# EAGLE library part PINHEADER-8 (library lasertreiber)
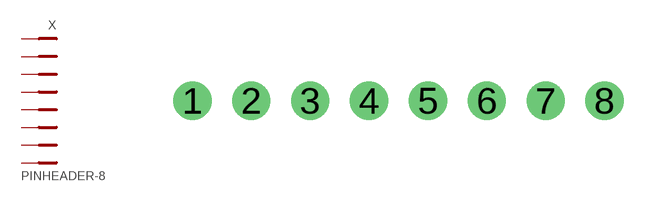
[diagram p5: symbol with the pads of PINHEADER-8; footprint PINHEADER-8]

Designator prefix X

## PINHEADER-8  [PINHEADER-8]
1  1
2  2
3  3
4  4
5  5
6  6
7  7
8  8

## Footprint PINHEADER-8 (pad centres in mm)
drill 1.1: 1 -8.89,0; 2 -6.35,0; 3 -3.81,0; 4 -1.27,0; 5 1.27,0; 6 3.81,0; 7 6.35,0; 8 8.89,0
